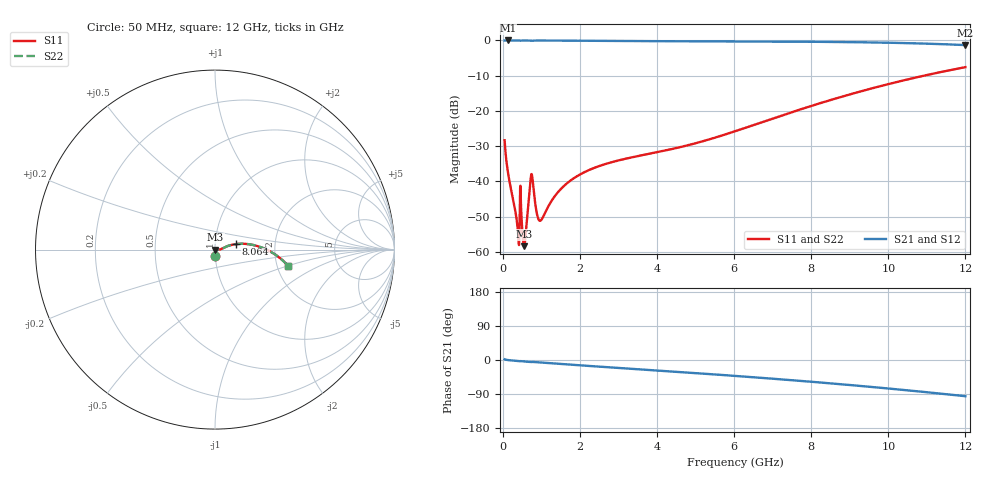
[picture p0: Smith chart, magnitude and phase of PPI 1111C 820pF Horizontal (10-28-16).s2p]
# MHz S MA R 50
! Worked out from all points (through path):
!   1601 points, 50 MHz to 12 GHz, reference 50 ohm
!   highest |S21| = 0.00 dB at 139.6 MHz (marker M1); lowest = -1.3 dB at 12 GHz (marker M2)
!   group delay of S21, straight-line fit = 21.5 ps
!   lowest |S11| = -58.4 dB at 557.9 MHz (marker M3), VSWR 1.00, Z = 50.1 - j0.0171 ohm
!   |S11| at or under -10 dB: start of sweep to 10.93 GHz
!   |S22| runs from -58.4 to -7.6 dB; largest |S21 - S12| = 0
!   S11 on the Smith chart (normalised r, x): 50 MHz: 1.00, -0.08; 8.064 GHz: 1.26, +0.08; 12 GHz: 2.30, -0.50
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50  0.03835 -87.7  0.999 1.9  0.999 1.9  0.03835 -87.7
139.625  0.01309 -88.2  0.9995 -0.2  0.9995 -0.2  0.01309 -88.2
311.4062  0.004279 -83.1  0.9993 -1.9  0.9993 -1.9  0.004279 -83.1
371.1562  0.002625 -75.4  0.9992 -2.4  0.9992 -2.4  0.002625 -75.4
423.4375  0.001248 -19.4  0.9988 -2.9  0.9988 -2.9  0.001248 -19.4
498.125  0.002482 -64.8  0.9988 -3.3  0.9988 -3.3  0.002482 -64.8
557.875  0.001205 -8.1  0.9988 -3.8  0.9988 -3.8  0.001205 -8.1
602.6875  0.001948 35.4  0.9985 -4.2  0.9985 -4.2  0.001948 35.4
699.7812  0.007595 41.7  0.9947 -5.1  0.9947 -5.1  0.007595 41.7
744.5938  0.01268 4.2  0.9874 -5.2  0.9874 -5.2  0.01268 4.2
789.4062  0.008931 -37.6  0.9924 -5.1  0.9924 -5.1  0.008931 -37.6
901.4375  0.003215 -31.3  0.997 -6.1  0.997 -6.1  0.003215 -31.3
983.5938  0.002778 -2.9  0.9972 -6.8  0.9972 -6.8  0.002778 -2.9
1461.594  0.007316 29.7  0.9943 -10.3  0.9943 -10.3  0.007316 29.7
2044.156  0.01287 18.1  0.989 -14.3  0.989 -14.3  0.01287 18.1
2783.562  0.01844 5.3  0.983 -19.3  0.983 -19.3  0.01844 5.3
4038.312  0.02621 0.1  0.9765 -27.8  0.9765 -27.8  0.02621 0.1
6025  0.05141 12.9  0.9692 -41.9  0.9692 -41.9  0.05141 12.9
8019.156  0.1184 14.8  0.9573 -57.5  0.9573 -57.5  0.1184 14.8
8063.969  0.1205 14.7  0.9569 -57.9  0.9569 -57.9  0.1205 14.7
10013.31  0.2409 4.4  0.928 -75.3  0.928 -75.3  0.2409 4.4
12000  0.4173 -12.5  0.8591 -95.5  0.8591 -95.5  0.4173 -12.5
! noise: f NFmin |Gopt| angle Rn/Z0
50  0.0003803  0.8687  0.365  0.0006234
1372  0.00792  0.8315  9.386  0.009846
2701  0.02013  0.8691  18.35  0.03225
4031  0.02909  0.8686  27.07  0.04501
5360  0.03609  0.8645  35.46  0.0519
6682  0.04227  0.8623  43.4  0.05685
8012  0.04826  0.8626  50.95  0.06145
9341  0.05434  0.8653  58.03  0.06636
1.067e+04  0.06074  0.8701  64.65  0.07201
1.2e+04  0.06769  0.8764  70.8  0.07881
